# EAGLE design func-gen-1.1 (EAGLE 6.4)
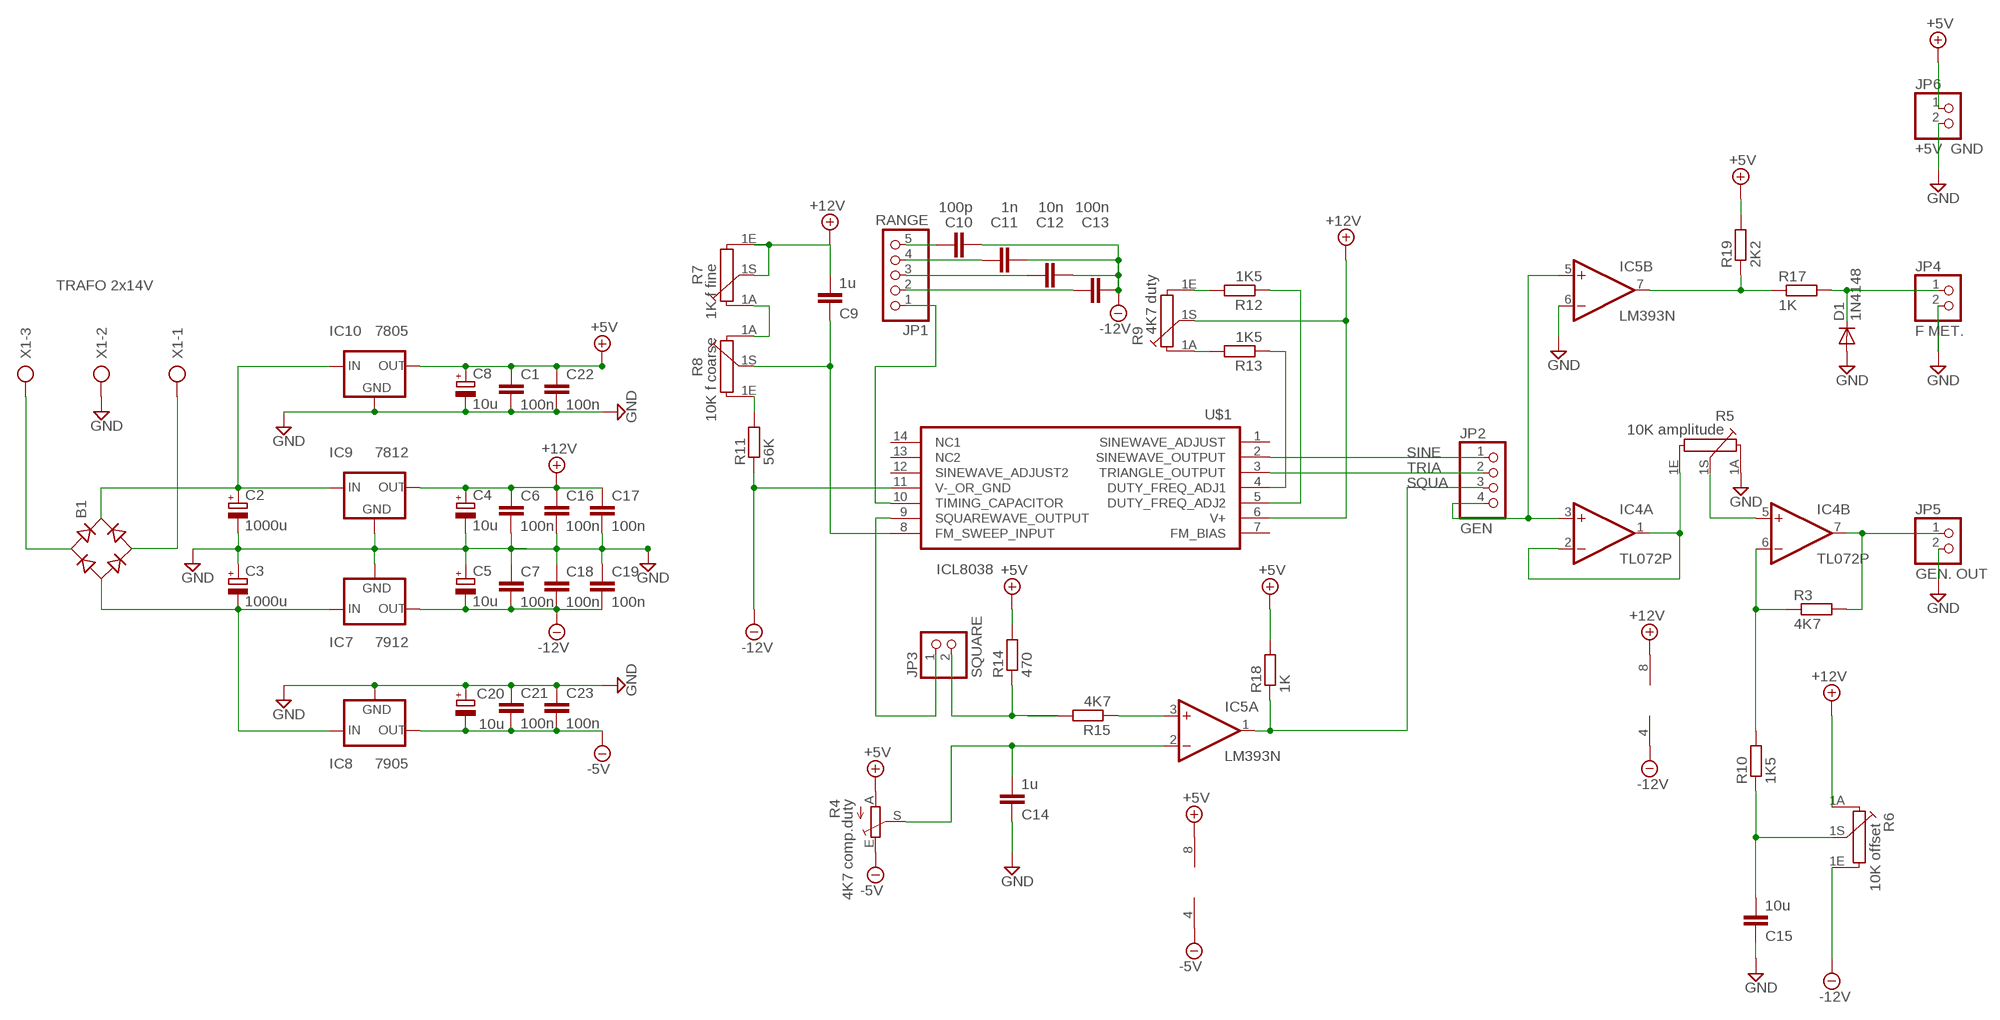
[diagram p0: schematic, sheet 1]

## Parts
B1  B-DIL  [B-DIL]
C1  100n  C-EU050-025X075  [C050-025X075]
C2  1000u  CPOL-EUE5-10.5  [E5-10,5]
C3  1000u  CPOL-EUE5-10.5  [E5-10,5]
C4  10u  CPOL-EUE2.5-6  [E2,5-6]
C5  10u  CPOL-EUE2.5-6  [E2,5-6]
C6  100n  C-EU050-025X075  [C050-025X075]
C7  100n  C-EU050-025X075  [C050-025X075]
C8  10u  CPOL-EUE2.5-6  [E2,5-6]
C9  1u  C-EU050-025X075  [C050-025X075]
C10  100p  C-EU050-025X075  [C050-025X075]
C11  1n  C-EU050-025X075  [C050-025X075]
C12  10n  C-EU050-025X075  [C050-025X075]
C13  100n  C-EU050-025X075  [C050-025X075]
C14  1u  C-EU050-025X075  [C050-025X075]
C15  10u  C-EU050-025X075  [C050-025X075]
C16  100n  C-EU050-025X075  [C050-025X075]
C17  100n  C-EU050-025X075  [C050-025X075]
C18  100n  C-EU050-025X075  [C050-025X075]
C19  100n  C-EU050-025X075  [C050-025X075]
C20  10u  CPOL-EUE2.5-6  [E2,5-6]
C21  100n  C-EU050-025X075  [C050-025X075]
C22  100n  C-EU050-025X075  [C050-025X075]
C23  100n  C-EU050-025X075  [C050-025X075]
D1  1N4148  1N4148DO35-7  [DO35-7]
IC4  TL072P  [DIL08]
IC5  LM393N  [DIL08]
IC7  7912  79XXS  [79XXS]
IC8  7905  79XXS  [79XXS]
IC9  7812  78XXS  [78XXS]
IC10  7805  78XXS  [78XXS]
JP1  RANGE  PINHD-1X5  [1X05]
JP2  GEN  PINHD-1X4  [1X04]
JP3  SQUARE  PINHD-1X2  [1X02]
JP4  F MET.  PINHD-1X2  [1X02]
JP5  GEN. OUT  PINHD-1X2  [1X02]
JP6  +5V GND  PINHD-1X2  [1X02]
R3  4K7  R-EU_0204/7  [0204/7]
R4  4K7 comp.duty  TRIM_EU-CA9V  [CA9V]
R5  10K amplitude  PC16S  [PC16S]
R6  10K offset  PC16S  [PC16S]
R7  1K f fine  PC16S  [PC16S]
R8  10K f coarse  PC16S  [PC16S]
R9  4K7 duty  PC16S  [PC16S]
R10  1K5  R-EU_0207/10  [0207/10]
R11  56K  R-EU_0204/7  [0204/7]
R12  1K5  R-EU_0204/7  [0204/7]
R13  1K5  R-EU_0204/7  [0204/7]
R14  470  R-EU_0204/7  [0204/7]
R15  4K7  R-EU_0204/7  [0204/7]
R17  1K  R-EU_0204/7  [0204/7]
R18  1K  R-EU_0204/7  [0204/7]
R19  2K2  R-EU_0204/7  [0204/7]
U$1  ICL8038  [DIP14]
X1  AK500/3  [AK500/3]

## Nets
+5V: C1.1 C8.+ C22.1 IC5.8(P:V+) IC10.OUT JP6.1 R4.A R14.2 R18.2 R19.2
+12V: C4.+ C6.1 C9.2 C16.1 C17.1 IC4.8(P:V+) IC9.OUT R6.1A R7.1E R7.1S R9.1S U$1.6(V+)
-5V: C20.- C21.2 C23.2 IC5.4(P:V-) IC8.OUT R4.E
-12V: C5.- C7.2 C10.2 C11.2 C12.2 C13.2 C18.2 C19.2 IC4.4(P:V-) IC7.OUT R6.1E R11.1 U$1.11(V-_OR_GND)
GND: C1.2 C2.- C3.+ C4.- C5.+ C6.2 C7.1 C8.- C14.1 C15.1 C16.2 C17.2 C18.1 C19.1 C20.+ C21.1 C22.2 C23.1 D1.A IC5.6(B:-IN) IC7.GND IC8.GND IC9.GND IC10.GND JP4.2 JP5.2 JP6.2 R5.1A X1.2
N$1: C9.1 R8.1S U$1.8(FM_SWEEP_INPUT)
N$2: B1.AC1 X1.3
N$3: B1.AC2 X1.1
N$4: B1.+ C2.+ IC9.IN IC10.IN
N$5: B1.- C3.- IC7.IN IC8.IN
N$6: JP1.1 U$1.10(TIMING_CAPACITOR)
N$7: C13.1 JP1.2
N$8: C12.1 JP1.3
N$9: C11.1 JP1.4
N$10: C10.1 JP1.5
N$11: IC4.3(A:+IN) IC5.5(B:+IN) JP2.4
N$13: IC4.1(A:OUT) IC4.2(A:-IN) R5.1E
N$14: JP3.1 U$1.9(SQUAREWAVE_OUTPUT)
N$15: IC4.5(B:+IN) R5.1S
N$16: C15.2 R6.1S R10.1
N$17: IC4.6(B:-IN) R3.1 R10.2
N$18: IC4.7(B:OUT) JP5.1 R3.2
N$19: R7.1A R8.1A
N$20: R8.1E R11.2
N$21: R9.1E R12.2
N$22: R9.1A R13.2
N$23: R13.1 U$1.4(DUTY_FREQ_ADJ1)
N$24: R12.1 U$1.5(DUTY_FREQ_ADJ2)
N$25: JP3.2 R14.1 R15.2
N$26: C14.2 IC5.2(A:-IN) R4.S
N$27: IC5.7(B:OUT) R17.1 R19.1
N$29: D1.C JP4.1 R17.2
N$30: IC5.3(A:+IN) R15.1
SINE: JP2.1 U$1.2(SINEWAVE_OUTPUT)
SQUA: IC5.1(A:OUT) JP2.3 R18.1
TRIA: JP2.2 U$1.3(TRIANGLE_OUTPUT)
Unconnected: U$1.1(SINEWAVE_ADJUST) U$1.7(FM_BIAS) U$1.12(SINEWAVE_ADJUST2) U$1.13(NC2) U$1.14(NC1)

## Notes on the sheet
- TRAFO 2x14V

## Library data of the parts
B1 = rectifier:B-DIL: RECTIFIER
C1 C6 C7 C9-C19 C21-C23 = rcl:C-EU: CAPACITOR, European symbol
C2-C5 C8 C20 = rcl:CPOL-EU: POLARIZED CAPACITOR, European symbol
D1 = diode:1N4148: DIODE
IC4 = linear:TL072: OP AMP
IC5 = linear:LM393: COMPARATOR
IC7 IC8 = v-reg-3:79XXS: VOLTAGE REGULATOR
IC9 IC10 = v-reg-3:78XXS: VOLTAGE REGULATOR
JP1 = pinhead:PINHD-1X5: PIN HEADER
JP2 = pinhead:PINHD-1X4: PIN HEADER
JP3-JP6 = pinhead:PINHD-1X2: PIN HEADER
R3 R10-R15 R17-R19 = rcl:R-EU_: RESISTOR, European symbol
R4 = pot:TRIM_EU-: POTENTIOMETER
R5-R9 = piher:PC16S: POTENTIOMETER single carbon potentiometer, 16 mm, S3ROH
U$1 = GuShH:ICL8038
X1 = con-ptr500:AK500/3: CONNECTOR

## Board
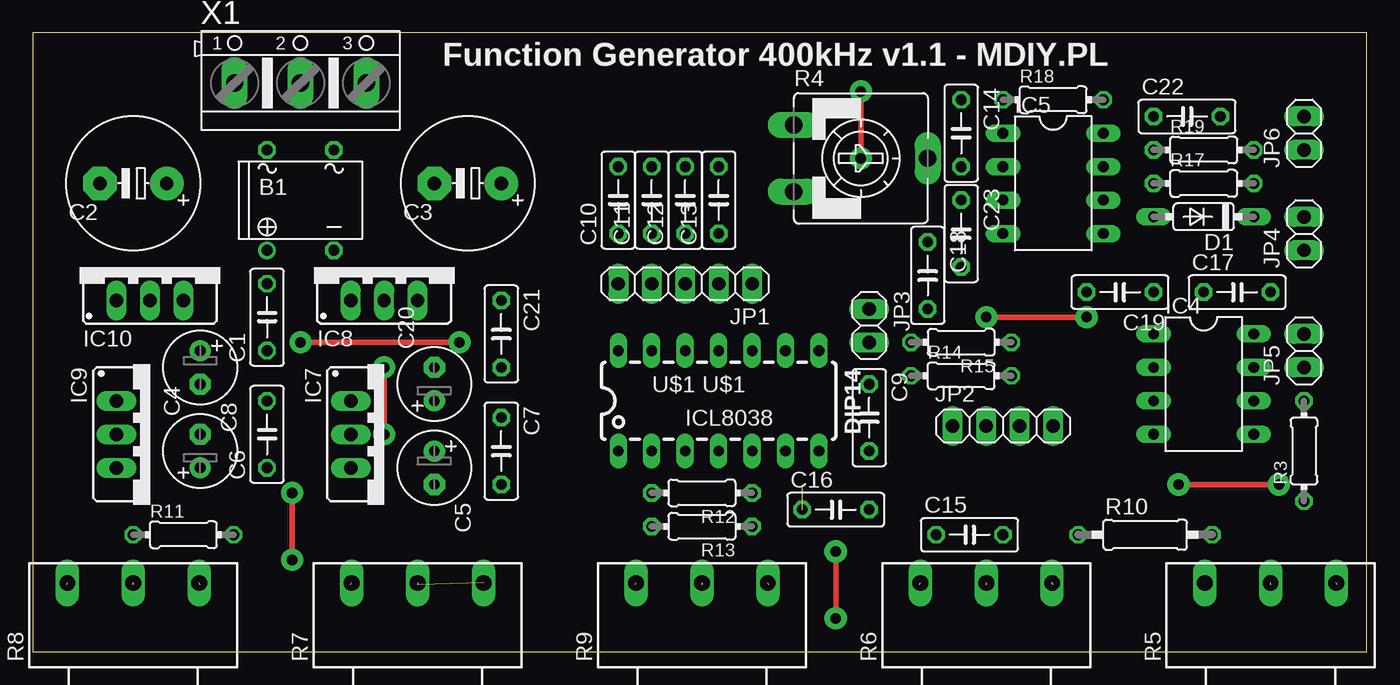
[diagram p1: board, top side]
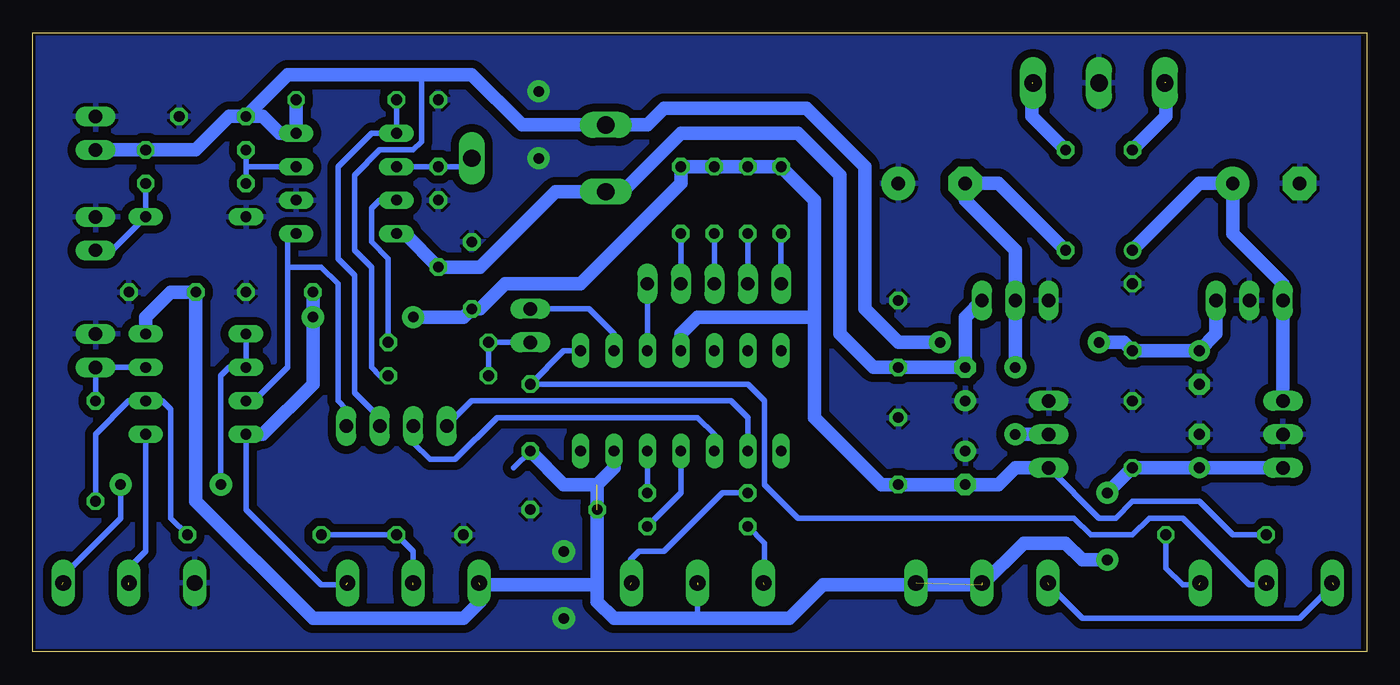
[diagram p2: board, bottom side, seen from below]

Size 101.27 x 46.98 mm. Coordinates in mm from the lower left corner, seen from the top.
Outline: 0,0 101.27,0 101.27,46.98 0,46.98 0,0
Copper layers (1*16): Top 0.035mm / dielectric 1.5mm / Bottom 0.035mm
Design rules "default *": minimum track width 10mil, minimum drill 24mil, track to track 24mil, track to pad 24mil, pad to pad 8mil, via to via 8mil, smd to smd 8mil, copper to edge 8mil, drill to drill 8mil, minimum pad ring 10mil, minimum via ring 8mil, stop-mask expansion 4mil, vias tented up to drill 0mil, thermal gap 10mil

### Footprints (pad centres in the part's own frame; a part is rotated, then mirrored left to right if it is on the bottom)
B-DIL = drill 0.813: + -2.54,-3.81 | drill 0.813 octagon: - 2.54,-3.81; AC1 2.54,3.81; AC2 -2.54,3.81
C050-025X075 = drill 0.813 octagon: 1 -2.54,0; 2 2.54,0
E5-10,5 = drill 1.016 pad 2.54: + -2.54,0 | drill 1.016 pad 2.54 octagon: - 2.54,0
E2,5-6 = drill 0.813 pad 1.6: + -1.27,0 | drill 0.813 pad 1.6 octagon: - 1.27,0
DO35-7 = drill 0.813 long: A 3.81,0; C -3.81,0
DIL08 = drill 0.813 long: 1 -3.81,-3.81; 2 -1.27,-3.81; 3 1.27,-3.81; 4 3.81,-3.81; 5 3.81,3.81; 6 1.27,3.81; 7 -1.27,3.81; 8 -3.81,3.81
79XXS = drill 1.016 long: GND -2.54,-2.54; IN 0,-2.54; OUT 2.54,-2.54
78XXS = drill 1.016 long: GND 0,-2.54; IN -2.54,-2.54; OUT 2.54,-2.54
1X05 = drill 1.016 long: 1 -5.08,0; 2 -2.54,0; 3 0,0; 4 2.54,0; 5 5.08,0
1X04 = drill 1.016 long: 1 -3.81,0; 2 -1.27,0; 3 1.27,0; 4 3.81,0
1X02 = drill 1.016 long: 1 -1.27,0; 2 1.27,0
0204/7 = drill 0.813 octagon: 1 -3.81,0; 2 3.81,0
CA9V = drill 1.321 long: A -2.54,-5.08; E 2.54,-5.08; S 0,5.08
PC16S = drill 1.2 long: 1A -5,6.5; 1E 5,6.5; 1S 0,6.5
0207/10 = drill 0.813 octagon: 1 -5.08,0; 2 5.08,0
DIP14 = drill 0.813 long: 1 -7.62,-3.81; 2 -5.08,-3.81; 3 -2.54,-3.81; 4 0,-3.81; 5 2.54,-3.81; 6 5.08,-3.81; 7 7.62,-3.81; 8 7.62,3.81; 9 5.08,3.81; 10 2.54,3.81; 11 0,3.81; 12 -2.54,3.81; 13 -5.08,3.81; 14 -7.62,3.81
AK500/3 = drill 1.321 long: 1 -5.004,0; 2 0,0; 3 5.004,0

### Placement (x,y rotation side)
B1  20.32,34.29 0 top
C1  17.78,25.4 90 top
C2  7.62,35.56 180 top
C3  33.02,35.56 180 top
C4  12.7,15.24 90 top
C5  30.48,13.97 270 top
C6  17.78,16.51 90 top
C7  35.56,15.24 270 top
C8  12.7,21.59 270 top
C9  63.5,17.78 270 top
C10  44.45,34.29 90 top
C11  46.99,34.29 90 top
C12  49.53,34.29 90 top
C13  52.07,34.29 90 top
C14  70.48,39.37 270 top
C15  71.12,8.89 0 top
C16  60.96,10.8 0 top
C17  91.44,27.3 0 top
C18  67.94,28.57 270 top
C19  82.55,27.3 180 top
C20  30.48,20.32 90 top
C21  35.56,24.13 270 top
C22  87.63,40.64 0 top
C23  70.48,31.75 270 top
D1  88.9,33.02 180 top
IC4  88.9,20.32 270 top
IC5  77.47,35.56 270 top
IC7  26.67,16.51 270 top
IC8  26.67,29.21 0 top
IC9  8.89,16.51 270 top
IC10  8.89,29.21 0 top
JP1  49.53,27.94 180 top
JP2  73.66,17.14 0 top
JP3  63.5,24.77 270 top
JP4  96.52,31.75 90 top
JP5  96.52,22.86 90 top
JP6  96.52,39.37 90 top
R3  96.52,15.24 90 top
R4  62.87,37.47 270 top
R5  93.98,-1.27 0 top
R6  72.39,-1.27 0 top
R7  29.21,-1.27 0 top
R8  7.62,-1.27 0 top
R9  50.8,-1.27 0 top
R10  84.45,8.89 0 top
R11  11.43,8.89 0 top
R12  50.8,12.07 180 top
R13  50.8,9.52 180 top
R14  70.48,20.96 0 top
R15  70.48,23.5 180 top
R17  88.9,35.56 0 top
R18  77.47,41.91 0 top
R19  88.9,38.1 0 top
U$1  52.07,19.05 0 top
X1  20.32,43.18 0 top

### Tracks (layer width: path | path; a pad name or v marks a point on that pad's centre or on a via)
+5V  (via drill 0.8 pad 1.68)
  Top 0.406: v20.32,23.5 v32.38,23.5
  Bottom 0.406: R14.2 74.93,20.96 75.56,21.59 75.56,29.21 76.83,30.48 76.83,36.2 74.93,38.1 72.39,38.1 71.75,38.73 71.75,43.81
  Bottom 1.016: JP6.1 R19.2 88.9,38.1 86.36,40.64 C22.1 | C22.1 83.82,40.64 82.55,39.37 IC5.8 R18.2 | C22.1 81.91,43.81 71.75,43.81 67.94,43.81 64.14,40.01 R4.A 54.61,40.01 53.34,41.27 42.55,41.27 38.1,36.83 38.1,26.04 35.56,23.5 v32.38,23.5 | v20.32,23.5 18.41,23.5 C1.1 C8.+ 11.43,24.13 IC10.OUT
+12V  (via drill 0.8 pad 1.68)  (5 unrouted)
  Top 0.406: v19.68,12.07 v19.68,6.99
  Bottom 0.406: 50.8,2.54 50.8,5.08 | C9.2 64.77,13.97
  Bottom 1.016: U$1.6 57.15,13.97 58.42,12.7 | 58.42,12.7 58.42,5.08 | 58.42,5.08 58.42,3.81 57.15,2.54 50.8,2.54 43.82,2.54 41.28,5.08 29.21,5.08 26.04,8.25 22.86,8.25 21.59,6.99 v19.68,6.99 | 58.42,5.08 67.31,5.08 67.31,3.81 68.58,2.54 80.01,2.54 88.9,11.43 C17.1 90.8,27.3 92.71,25.4 IC4.8 | 58.42,12.7 60.96,12.7 C9.2 | v19.68,12.07 C6.1 C4.+ IC9.OUT
-5V
  Bottom 1.016: IC5.4 73.02,31.75 C23.2 67.31,29.21 61.6,34.93 R4.E 56.52,34.93 52.07,39.37 43.18,39.37 40.01,36.2 40.01,24.13 37.47,21.59 C21.2 C20.- 30.48,25.4 IC8.OUT
-12V  (via drill 0.8 pad 1.68)  (1 unrouted)
  Top 0.406: v72.39,25.4 v80.01,25.4
  Bottom 0.406: IC4.4 85.09,10.8 79.38,5.08 77.47,5.08 | R11.1 10.16,8.89 12.7,11.43 17.78,11.43 19.05,10.16 20.32,10.16 IC7.OUT
  Bottom 1.016: 41.91,25.4 50.8,25.4 52.07,24.13 U$1.11 | 41.91,25.4 41.91,34.29 C10.2 C11.2 C12.2 C13.2 52.07,35.56 59.69,27.94 65.41,27.94 67.31,26.04 C18.2 68.58,25.4 v72.39,25.4 | IC4.4 83.82,16.51 80.01,20.32 v80.01,25.4 C19.2 | 41.91,25.4 41.91,17.78 36.83,12.7 C7.2 C5.- 27.94,12.7 26.67,13.97 IC7.OUT
GND  (via drill 0.8 pad 1.68)
  Top 0.406: v60.96,7.62 v60.96,2.54 | v62.87,42.55 v62.87,37.47
  pour Bottom: 0.64,46.99 100.96,46.99 100.96,0 0.64,0
N$1  (1 unrouted)
  Bottom 0.406: U$1.8 60.96,22.86 C9.1 46.99,20.32 45.72,19.05 45.72,12.7 43.18,10.16 22.22,10.16 20.95,8.89 17.78,8.89 16.51,10.16 13.97,10.16 8.89,5.08 7.62,5.08
N$2  (1 unrouted)
  Bottom 1.016: 25.4,43.18 25.4,40.64 B1.AC1
N$3  (1 unrouted)
  Bottom 1.016: 15.24,43.18 15.24,40.64 B1.AC2
N$4
  Bottom 1.016: B1.+ 12.7,35.56 C2.+ 10.16,31.75 6.35,27.94 IC10.IN IC9.IN
N$5  (via drill 0.8 pad 1.68)
  Top 0.406: v26.67,21.59 v26.67,16.51
  Bottom 1.016: B1.- 27.94,35.56 C3.- 30.48,34.29 26.67,30.48 IC8.IN v26.67,21.59 | IC7.IN v26.67,16.51
N$6
  Bottom 0.406: JP1.1 U$1.10
N$7
  Bottom 0.406: C13.1 JP1.2
N$8
  Bottom 0.406: C12.1 JP1.3
N$9
  Bottom 0.406: C11.1 JP1.4
N$10
  Bottom 0.406: C10.1 JP1.5
N$11
  Bottom 0.406: IC4.3 84.45,19.05 81.91,21.59 81.91,31.12 | 81.91,31.12 IC5.5 81.91,31.12 | 81.91,31.12 81.91,29.21 79.38,29.21 78.1,27.94 78.1,19.05 77.47,18.41 JP2.4
N$13  (via drill 0.8 pad 1.68)  (1 unrouted)
  Top 0.406: v86.99,12.7 v94.61,12.7
  Bottom 0.406: IC4.1 IC4.2 86.36,21.59 86.99,20.96 v86.99,12.7 | v94.61,12.7 94.61,10.16 99.06,5.72 99.06,5.08
N$14
  Bottom 0.406: JP3.1 59.05,26.04 57.15,24.13 U$1.9
N$15  (1 unrouted)
  Bottom 0.406: IC4.5 92.71,7.62 93.98,6.35 93.98,5.08
N$16  (1 unrouted)
  Bottom 0.406: R10.1 C15.2 72.39,7.62 72.39,5.08
N$17
  Bottom 0.406: R3.1 96.52,16.51 93.98,19.05 IC4.6 91.44,19.05 90.8,18.41 90.8,10.16 R10.2
N$18
  Bottom 0.406: IC4.7 JP5.1 R3.2
N$19  (2 unrouted)
  Bottom 0.406: 24.13,5.08 21.59,2.54 5.08,2.54 2.54,5.08
N$20  (1 unrouted)
  Bottom 0.406: R11.2 15.24,6.35 13.97,5.08 12.7,5.08
N$21  (1 unrouted)
  Bottom 0.406: R12.2 48.9,12.07 53.34,7.62 55.25,7.62 55.88,6.99 55.88,5.08
N$22  (1 unrouted)
  Bottom 0.406: R13.2 45.72,8.25 45.72,5.08
N$23
  Bottom 0.406: U$1.4 52.07,12.07 R13.1
N$24
  Bottom 0.406: U$1.5 R12.1
N$25
  Bottom 0.406: JP3.2 R15.2 R14.1
N$26
  Bottom 0.406: R4.S 68.58,36.83 C14.2 IC5.2
N$27
  Bottom 0.406: IC5.7 85.09,36.83 R17.1 R19.1
N$29
  Bottom 0.406: JP4.1 95.25,30.48 D1.C R17.2
N$30
  Bottom 0.406: R15.1 74.3,29.84 75.56,31.12 75.56,33.66 74.93,34.29 IC5.3
SINE
  Bottom 0.406: U$1.2 46.99,17.78 48.26,19.05 67.94,19.05 JP2.1
SQUA
  Bottom 0.406: JP2.3 74.93,17.78 76.83,19.69 76.83,28.57 78.1,29.84 78.1,36.83 75.56,39.37 IC5.1 R18.1
TRIA
  Bottom 0.406: JP2.2 72.39,15.88 71.12,14.61 69.21,14.61 66.04,17.78 50.8,17.78 49.53,16.51 U$1.3

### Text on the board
tPlace: Function Generator 400kHz v1.1 - MDIY.PL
